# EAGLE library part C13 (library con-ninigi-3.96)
NINIGI
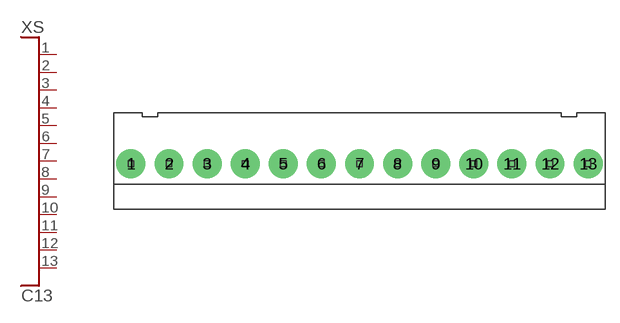
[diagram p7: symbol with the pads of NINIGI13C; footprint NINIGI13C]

Designator prefix XS

## C13  [NINIGI13C]
1  P$1
2  P$2
3  P$3
4  P$4
5  P$5
6  P$6
7  P$7
8  P$8
9  P$9
10  P$10
11  P$11
12  P$12
13  P$13

## Footprint NINIGI13C (pad centres in mm)
drill 1.6 pad 3: 1 -23.76,0; 2 -19.8,0; 3 -15.84,0; 4 -11.88,0; 5 -7.92,0; 6 -3.96,0; 7 0,0; 8 3.96,0; 9 7.92,0; 10 11.88,0; 11 15.84,0; 12 19.8,0; 13 23.76,0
